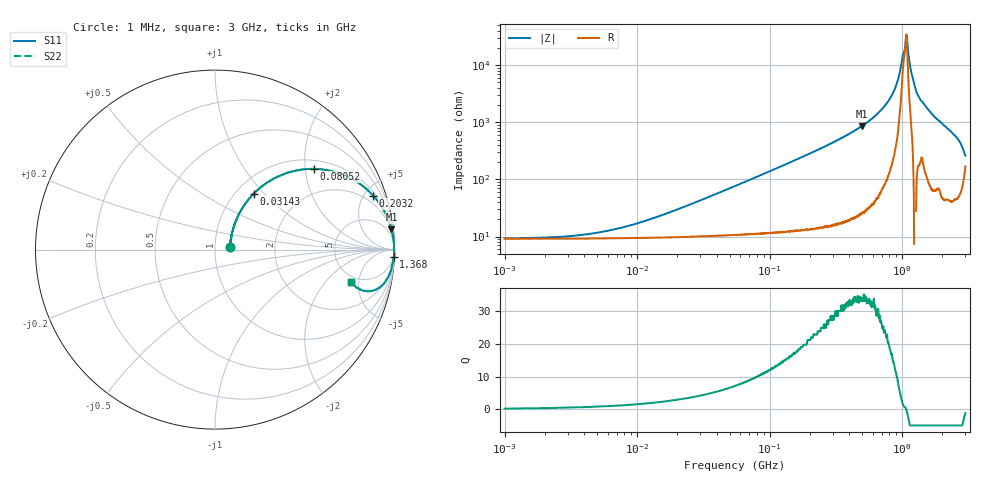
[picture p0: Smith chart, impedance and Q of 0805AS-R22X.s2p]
!s-Parameter Generated by FASTRON Sdn. Bhd.
!FASTRON P/N : 0805AS-R22X
!Keysight Technologies: E4991B_MY54100416_A.01.15
!Date: Mon Jun 15 12:53:01 2026
!Version  :Rev01  Mon Jun 15 12:53:01 2026
!Data & Calibration Information:
!Freq  S11  S21  S12  S22
!PortZ  Port1:50+j0  Port2:50+j0
!When reading reference impedance value at option line is always used.
! Remarks : This data is being provided solely for informational purposes.
# Hz S dB R 50
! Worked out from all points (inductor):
!   1601 points, 1 MHz to 3 GHz, reference 50 ohm
!   read as one part in series: L = 222 nH near 20.96 MHz
!   highest Q = 34.3 at 495.2 MHz (marker M1), where L = 277 nH
!   self-resonance near 1.07 GHz
!   S11 on the Smith chart (normalised r, x): 1 MHz: 1.18, +0.03; 31.43 MHz: 1.20, +0.88; 80.52 MHz: 1.22, +2.23; 203.2 MHz: 1.28, +5.77; 1.368 GHz: 5, -50; 3 GHz: 4.37, -3.95
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1000000  -21.40 8.1  -0.76 -0.8  -0.76 -0.8  -21.40 8.1
3804036  -20.20 27.6  -0.78 -2.8  -0.78 -2.8  -20.20 27.6
1.447069e7  -13.90 54.3  -0.94 -10.5  -0.94 -10.5  -13.90 54.3
3.142935e7  -8.41 55.3  -1.48 -21.7  -1.48 -21.7  -8.41 55.3
5.504702e7  -4.83 47.5  -2.57 -34.6  -2.57 -34.6  -4.83 47.5
8.051876e7  -2.96 39.2  -3.94 -45.1  -3.94 -45.1  -2.96 39.2
2.032073e8  -0.62 18.8  -9.81 -68.5  -9.81 -68.5  -0.62 18.8
2.083556e8  -0.59 18.4  -10.00 -69.0  -10.00 -69.0  -0.59 18.4
4.951867e8  -0.09 6.6  -18.80 -81.7  -18.80 -81.7  -0.09 6.6
6.488164e8  -0.04 4.1  -23.00 -84.0  -23.00 -84.0  -0.04 4.1
7.925923e8  -0.03 2.4  -27.70 -84.8  -27.70 -84.8  -0.03 2.4
9.209708e8  -0.02 1.1  -34.30 -82.8  -34.30 -82.8  -0.02 1.1
1.0437e9  -0.04 0.2  -45.40 -33.5  -45.40 -33.5  -0.04 0.2
1.064802e9  -0.03 0.1  -49.20 -17.7  -49.20 -17.7  -0.03 0.1
1.10276e9  -0.02 -0.2  -46.30 62.2  -46.30 62.2  -0.02 -0.2
1.165162e9  -0.02 -0.7  -38.10 81.6  -38.10 81.6  -0.02 -0.7
1.237271e9  -0.00 -1.3  -33.10 89.1  -33.10 89.1  -0.00 -1.3
1.367504e9  -0.03 -2.2  -28.10 83.4  -28.10 83.4  -0.03 -2.2
1.76507e9  -0.06 -4.6  -21.90 82.5  -21.90 82.5  -0.06 -4.6
2.556106e9  -0.26 -10.0  -15.10 75.3  -15.10 75.3  -0.26 -10.0
2.783064e9  -0.53 -13.0  -12.90 68.5  -12.90 68.5  -0.53 -13.0
3e9  -2.17 -13.2  -10.50 36.4  -10.50 36.4  -2.17 -13.2
